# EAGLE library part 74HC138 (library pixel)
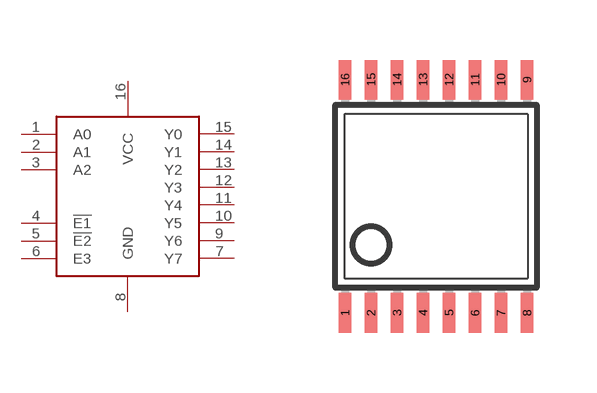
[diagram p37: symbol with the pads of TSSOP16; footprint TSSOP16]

Designator prefix -

## 74HC138  [TSSOP16]
1  A0
2  A1
3  A2
4  !E1
5  !E2
6  E3
7  Y7
8  GND
9  Y6
10  Y5
11  Y4
12  Y3
13  Y2
14  Y1
15  Y0
16  VCC

## Footprint TSSOP16 (pad centres in mm)
Thin Shrink Small Outline Plastic 16 MAX3223-MAX3243.pdf
smd 0.305 x 0.991: 1 -2.275,-2.918; 2 -1.625,-2.918; 3 -0.975,-2.918; 4 -0.325,-2.918; 5 0.325,-2.918; 6 0.975,-2.918; 7 1.625,-2.918; 8 2.275,-2.918; 9 2.275,2.918; 10 1.625,2.918; 11 0.975,2.918; 12 0.325,2.918; 13 -0.325,2.918; 14 -0.975,2.918; 15 -1.625,2.918; 16 -2.275,2.918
